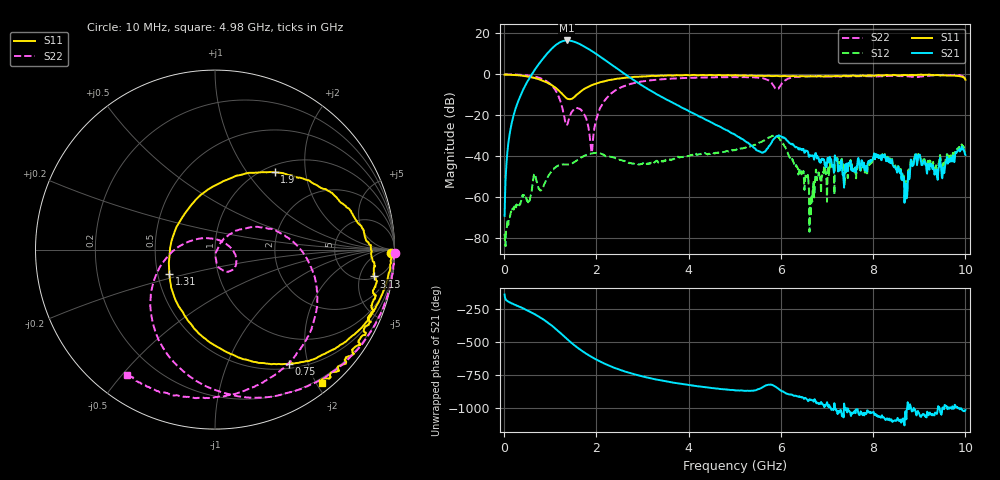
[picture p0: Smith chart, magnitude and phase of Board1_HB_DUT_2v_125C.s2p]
! Created Tue May 27 14:56:41 2025
# hz S ma R 50
! 2 Port Network Data from SP1.SP block
! freq  magS11  angS11  magS21  angS21  magS12  angS12  magS22  angS22
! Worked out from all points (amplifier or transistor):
!   1000 points, 10 MHz to 10 GHz, reference 50 ohm
!   highest |S21| = 16.6 dB at 1.36 GHz (marker M1)
!   |S21| within 3 dB of that: 1.079 GHz to 1.741 GHz (661.3 MHz wide, 46.9 % of centre)
!   unconditionally stable (mu >= 1): 16.19 MHz to 48.08 MHz; 51.14 MHz to end of sweep
!   at 1.67 GHz: K = 8.72, MAG = 15.2 dB, |S12| = -40.8 dB
!   at 5.01 GHz: K = 23.28, MAG = -13.0 dB, |S12| = -37.0 dB
!   at 10 GHz: K = 494.15, MAG = -30.7 dB, |S12| = -37.9 dB
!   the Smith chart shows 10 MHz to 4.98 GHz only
!   S11 on the Smith chart (normalised r, x): 10 MHz: 54, -45; 750 MHz: 0.57, -1.70; 1.31 GHz: 0.58, -0.17; 1.9 GHz: 1.11, +1.36; 3.13 GHz: 5, -8; 4.98 GHz: 0.13, -2.08
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1e7  0.9782 -1.0  0.0003431 -142.9  0.0001244 90.9  1.004 -0.9
2e8  0.9655 -13.9  0.09481 145.9  0.0005107 80.4  0.9922 -18.4
7.5e8  0.7587 -57.0  1.768 50.4  0.001564 72.2  0.8283 -80.9
9.3e8  0.6308 -75.6  3.205 9.7  0.002781 116.7  0.6665 -110.3
1.09e9  0.4924 -97.7  4.884 -33.5  0.005079 101.1  0.4435 -143.9
1.19e9  0.3932 -116.9  5.914 -63.8  0.005897 88.2  0.2712 -170.8
1.31e9  0.2875 -152.2  6.668 -102.1  0.006217 76.1  0.08431 130.0
1.36e9  0.2556 -172.7  6.753 -117.9  0.006179 74.0  0.05755 62.3
1.51e9  0.2712 123.2  6.332 -162.7  0.00702 74.4  0.1374 -30.8
1.68e9  0.3938 80.4  5.209 153.1  0.009336 66.1  0.1304 -66.4
1.9e9  0.5434 52.4  3.723 104.8  0.01156 43.7  0.01212 -26.2
2.25e9  0.7121 27.2  2.004 43.6  0.009796 13.1  0.2826 26.0
2.6e9  0.8215 9.6  1.048 -2.7  0.007663 2.2  0.5159 -5.8
3.13e9  0.8978 -9.6  0.4269 -52.1  0.006511 14.5  0.7045 -41.7
3.34e9  0.9207 -15.8  0.3115 -67.7  0.006914 11.2  0.7448 -53.8
4.98e9  0.9515 -51.2  0.03437 -145.2  0.01406 -11.3  0.8531 -124.9
5.01e9  0.9576 -51.9  0.03302 -147.5  0.01412 -12.0  0.854 -126.0
5.92e9  0.9155 -71.2  0.03092 -128.7  0.03006 -101.3  0.4469 -146.8
6.67e9  0.8955 -92.3  0.01004 139.9  0.0008789 116.6  0.9075 -157.8
8.34e9  0.9419 -134.1  0.007071 -8.6  0.007397 -13.9  0.9132 166.7
8.7e9  0.9672 -140.7  0.001465 54.4  0.002176 48.5  0.8978 160.0
1e10  0.7377 -161.4  0.0106 64.9  0.01274 62.2  0.8411 151.8
